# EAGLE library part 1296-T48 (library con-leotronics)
1.27mm SINGLE ROW FEMALE SOCKET Source: http://www.leotronics.co.uk/Conexcon/Data%20Sheets/sec.%20A/1296ing.pdf
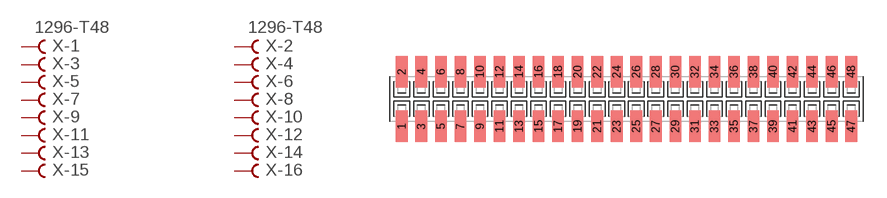
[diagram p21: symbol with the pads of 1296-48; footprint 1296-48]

Designator prefix X; gates -1=FVAL -2=FVAL -3=F -4=F -5=F -6=F -7=F -8=F -9=F -10=F -11=F -12=F -13=F -14=F -15=F -16=F -17=F -18=F -19=F -20=F -21=F -22=F -23=F -24=F -25=F -26=F -27=F -28=F -29=F -30=F -31=F -32=F -33=F -34=F -35=F -36=F -37=F -38=F -39=F -40=F -41=F -42=F -43=F -44=F -45=F -46=F -47=F -48=F

## 1296-T48 (OC_FARNELL: unknown; OC_NEWARK: unknown)  [1296-48]
1  -1:B  pas
2  -2:B  pas
3  -3:B  pas
4  -4:B  pas
5  -5:B  pas
6  -6:B  pas
7  -7:B  pas
8  -8:B  pas
9  -9:B  pas
10  -10:B  pas
11  -11:B  pas
12  -12:B  pas
13  -13:B  pas
14  -14:B  pas
15  -15:B  pas
16  -16:B  pas
17  -17:B  pas
18  -18:B  pas
19  -19:B  pas
20  -20:B  pas
21  -21:B  pas
22  -22:B  pas
23  -23:B  pas
24  -24:B  pas
25  -25:B  pas
26  -26:B  pas
27  -27:B  pas
28  -28:B  pas
29  -29:B  pas
30  -30:B  pas
31  -31:B  pas
32  -32:B  pas
33  -33:B  pas
34  -34:B  pas
35  -35:B  pas
36  -36:B  pas
37  -37:B  pas
38  -38:B  pas
39  -39:B  pas
40  -40:B  pas
41  -41:B  pas
42  -42:B  pas
43  -43:B  pas
44  -44:B  pas
45  -45:B  pas
46  -46:B  pas
47  -47:B  pas
48  -48:B  pas

## Footprint 1296-48 (pad centres in mm)
1.27mm SINGLE ROW FEMALE SOCKET Source: http://www.leotronics.co.uk/Conexcon/Data%20Sheets/sec.%20A/1296ing.pdf
smd 0.76 x 2.05: 1 -14.605,-1.78; 2 -14.605,1.78; 3 -13.335,-1.78; 4 -13.335,1.78; 5 -12.065,-1.78; 6 -12.065,1.78; 7 -10.795,-1.78; 8 -10.795,1.78; 9 -9.525,-1.78; 10 -9.525,1.78; 11 -8.255,-1.78; 12 -8.255,1.78; 13 -6.985,-1.78; 14 -6.985,1.78; 15 -5.715,-1.78; 16 -5.715,1.78; 17 -4.445,-1.78; 18 -4.445,1.78; 19 -3.175,-1.78; 20 -3.175,1.78; 21 -1.905,-1.78; 22 -1.905,1.78; 23 -0.635,-1.78; 24 -0.635,1.78; 25 0.635,-1.78; 26 0.635,1.78; 27 1.905,-1.78; 28 1.905,1.78; 29 3.175,-1.78; 30 3.175,1.78; 31 4.445,-1.78; 32 4.445,1.78; 33 5.715,-1.78; 34 5.715,1.78; 35 6.985,-1.78; 36 6.985,1.78; 37 8.255,-1.78; 38 8.255,1.78; 39 9.525,-1.78; 40 9.525,1.78; 41 10.795,-1.78; 42 10.795,1.78; 43 12.065,-1.78; 44 12.065,1.78; 45 13.335,-1.78; 46 13.335,1.78; 47 14.605,-1.78; 48 14.605,1.78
